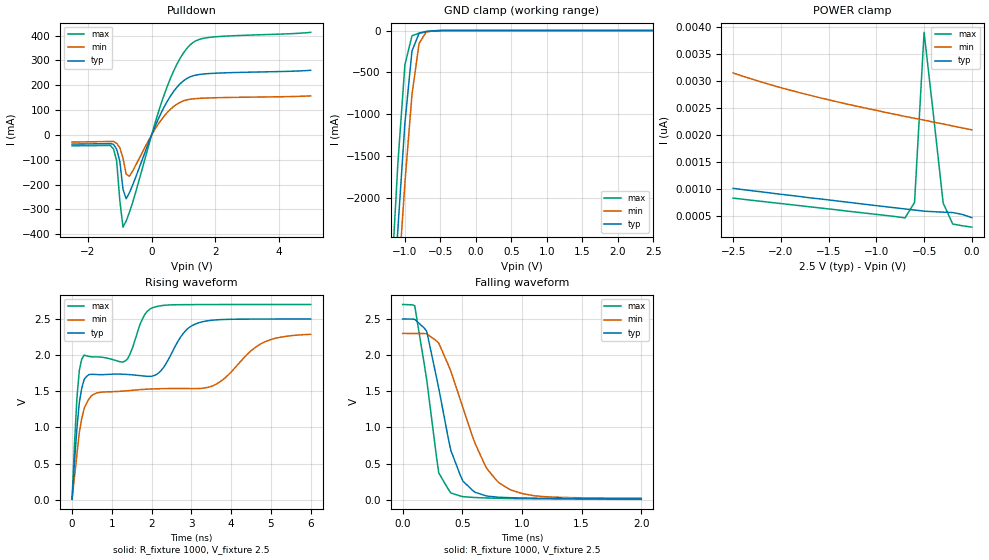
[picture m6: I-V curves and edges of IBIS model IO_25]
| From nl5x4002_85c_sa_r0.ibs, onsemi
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[Model]   IO_25
Model_type I/O_open_drain
Enable Active-High
Polarity Non-Inverting
Vinh=1.75
Vinl=0.75
Vref=2.5
Vmeas=1.25
Rref=1000
Cref=50p
C_comp   6.0p   NA   NA
[Model Spec]
Vinh   1.75   1.61   1.89
Vinl   0.75   0.69   0.81
Vmeas   1.25   1.15   1.35
[Temperature Range] 25   85   -40
[Voltage Range]   2.5   2.3   2.7
[POWER Clamp Reference]  2.5   2.3   2.7
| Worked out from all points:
|   slope of the pulldown table from 0 to 0.375 V, typ, clamps not added: 3.48 ohm
|   GND clamp passes 1 mA (typ) near -0.51 V on its own axis
|   falling waveform, R_fixture 1000, V_fixture 2.5: 20-80 % time 200ps typ, 304ps min, 135ps max; typ from 2.5 V to 0.013 V
|   rising waveform, R_fixture 1000, V_fixture 2.5: 20-80 % time 2.42ns typ, 4.02ns min, 1.51ns max; typ from 0.008 V to 2.5 V
[Pulldown]
-2.5V     -37.14mA   -28.84mA   -44mA
-1.2V     -37.75mA   -26.35mA   -56.23mA
-1.1V     -57.35mA   -33.83mA   -104mA
-1V       -105.9mA   -51.85mA   -264.7mA
-900mV    -218.8mA   -93.14mA   -371.5mA
-800mV    -257.2mA   -157.8mA   -346.4mA
-700mV    -233.7mA   -166.5mA   -312.5mA
400mV     114.1mA    76.63mA    163.7mA
800mV     192.6mA    124.2mA    285.9mA
1.2V      233.3mA    143.4mA    361.2mA
1.9V      247.7mA    149.2mA    393.8mA
5V        260.1mA    157mA      413mA
[GND Clamp]
-2.5V     -23.36A    -22.26A    -24.82A
-1.2V     -3.822A    -4.412A    -3.136A
-1.1V     -2.385A    -3.071A    -1.6A
-1V       -1.105A    -1.818A    -410.1mA
-900mV    -244.1mA   -763.4mA   -62.39mA
-800mV    -31.41mA   -154.3mA   -31.83mA
-700mV    -10.05mA   -17.99mA   -15.56mA
-500mV    -634.4uA   -553uA     -616uA
2.5V      463.5pA    2.096nA    287.2pA
[POWER Clamp]
-2.5V     1.008nA    3.153nA    826.2pA
-2.1V     919.6pA    2.93nA     745.4pA
-1.8V     856.2pA    2.784nA    685.7pA
-1.3V     750.1pA    2.571nA    583.9pA
-700mV    625.2pA    2.345nA    458.4pA
-600mV    605.1pA    2.31nA     745.8pA
-500mV    584.3pA    2.276nA    3.908nA
-400mV    573.9pA    2.239nA    2.341nA
-300mV    565.7pA    2.204nA    735.2pA
-200mV    558.1pA    2.167nA    345.2pA
-100mV    523.6pA    2.132nA    313.1pA
0V        463.3pA    2.096nA    286.8pA
[Falling Waveform]
R_fixture=1000
V_fixture=2.5
V_fixture_min=2.3
V_fixture_max=2.7
0s        2.5V       2.3V       2.7V
101ps     2.496V     2.299V     2.684V
202ps     2.33V      2.296V     1.658V
303ps     1.539V     2.165V     371.1mV
404ps     682.2mV    1.779V     94.5mV
505.1ps   259.2mV    1.275V     43.24mV
686.9ps   59.94mV    490.3mV    25.9mV
808.1ps   35.03mV    233.8mV    20.36mV
1.111ns   22.32mV    54.47mV    13.98mV
2ns       12.81mV    20.52mV    6.313mV
[Rising Waveform]
R_fixture=1000
V_fixture=2.5
V_fixture_min=2.3
V_fixture_max=2.7
0s        7.614mV    10.11mV    5.899mV
121.2ps   984.9mV    623.3mV    1.403V
181.8ps   1.344V     930.8mV    1.788V
303ps     1.664V     1.263V     2V
1.333ns   1.734V     1.505V     1.918V
1.818ns   1.71V      1.527V     2.554V
2.182ns   1.756V     1.535V     2.679V
3.152ns   2.441V     1.538V     2.699V
4.788ns   2.499V     2.169V     2.7V
6ns       2.5V       2.288V     2.7V
[Ramp]
R_load=1000
dV/dt_r   1.495E+0/1.457E-10   1.374E+0/1.265E-10   1.587E+0/1.490E-9
dV/dt_f   1.492E+0/1.999E-10   1.368E+0/3.025E-10   1.616E+0/1.345E-10
|[End   IO_25
